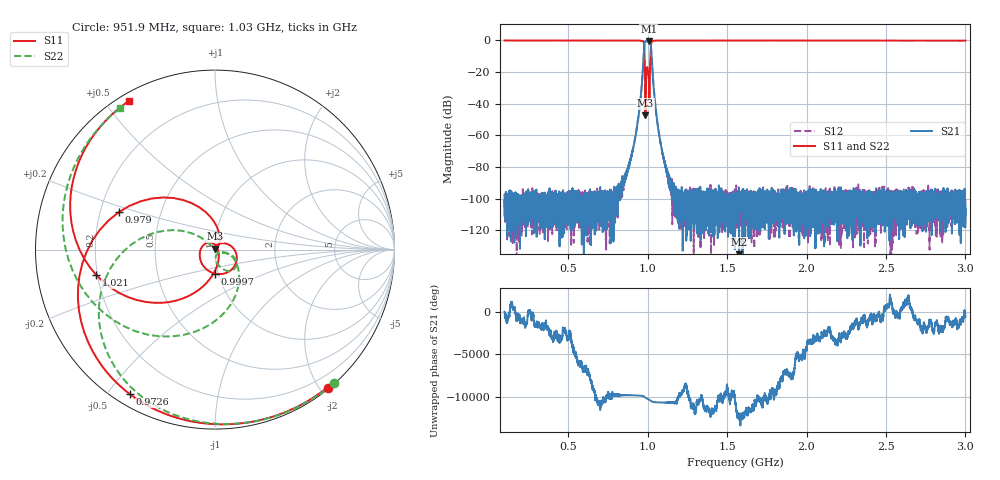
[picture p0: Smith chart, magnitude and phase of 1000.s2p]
# Hz S DB R 50
! Planar, S50180, 20087770, 20.1.2/1
! Date: 23.06.2021 14:41:15
! Data: Format (Calibration Info)
! Freq	S11:dB/Ang(F2)	S21:dB/Ang(F2)	S12:dB/Ang(F2)	S22:dB/Ang(F2)
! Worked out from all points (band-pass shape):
!   8991 points, 100 MHz to 3 GHz, reference 50 ohm
!   highest |S21| = -0.51 dB at 1.007 GHz (marker M1); lowest = -145.2 dB at 1.576 GHz (marker M2)
!   |S21| within 3 dB of the highest: 978.8 MHz to 1.021 GHz (42.07 MHz wide, 4.21 % of centre)
!   lowest |S11| = -47.2 dB at 986.5 MHz (marker M3), VSWR 1.01, Z = 50 + j0.436 ohm
!   |S11| at or under -10 dB: 981.1 MHz to 1.018 GHz (36.61 MHz wide, 3.66 % of centre)
!   |S22| runs from -48.1 to 0.0 dB; largest |S21 - S12| = 0.0024
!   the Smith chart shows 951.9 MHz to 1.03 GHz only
!   S11 on the Smith chart (normalised r, x): 951.9 MHz: 0.02, -2.11; 972.6 MHz: 0.04, -0.57; 979 MHz: 0.28, +0.17; 999.7 MHz: 0.96, -0.26; 1.021 GHz: 0.20, -0.10; 1.03 GHz: 0.03, +0.58
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1e8  0.02 154.2  -102.74 27.3  -105.04 -60.8  0.01 150.5
3.154839e8  -0.03 103.6  -104.06 -162.5  -105.95 113.6  -0.00 95.1
5.835484e8  -0.01 53.5  -99.00 93.9  -105.56 -126.6  0.01 44.5
8.725806e8  -0.00 -0.2  -83.11 -94.9  -81.66 -95.9  0.02 -5.7
9.13871e8  -0.02 -16.3  -65.95 -108.5  -65.75 -109.3  0.01 -19.6
9.519355e8  -0.07 -50.8  -40.45 -141.7  -40.44 -141.9  -0.04 -48.4
9.725806e8  -0.59 -120.5  -14.30 153.2  -14.30 153.1  -0.48 -104.7
9.790323e8  -4.79 158.9  -3.16 78.4  -3.16 78.2  -4.56 -169.9
9.864516e8  -47.19 86.0  -0.57 -30.8  -0.57 -30.9  -36.30 -49.5
9.996774e8  -17.51 -91.0  -0.55 -165.6  -0.55 -165.7  -16.79 -55.2
1.007097e9  -23.81 151.6  -0.51 122.2  -0.51 122.1  -22.27 -81.2
1.02129e9  -3.40 -167.8  -4.05 -59.5  -4.05 -59.6  -3.57 -139.9
1.029677e9  -0.38 120.0  -17.71 -144.5  -17.70 -144.7  -0.45 123.8
1.042258e9  -0.13 79.2  -34.54 169.1  -34.55 169.0  -0.14 73.8
1.066774e9  -0.06 47.9  -55.81 135.0  -55.76 135.4  -0.02 39.6
1.100968e9  -0.02 28.9  -74.52 117.3  -74.16 112.9  0.01 20.6
1.124839e9  -0.01 20.8  -84.09 106.2  -82.59 94.0  0.00 12.8
1.55e9  -0.01 -34.1  -105.67 -90.9  -103.65 -79.8  0.03 -38.7
1.575806e9  -0.01 -36.4  -145.17 170.6  -98.22 104.0  0.02 -40.8
2.033548e9  -0.04 -73.1  -97.86 -175.7  -97.78 89.2  -0.01 -74.4
2.516774e9  -0.07 -108.5  -97.96 -137.7  -98.17 -42.4  -0.05 -106.9
3e9  -0.11 -145.0  -106.63 117.5  -114.41 14.2  -0.09 -140.6
